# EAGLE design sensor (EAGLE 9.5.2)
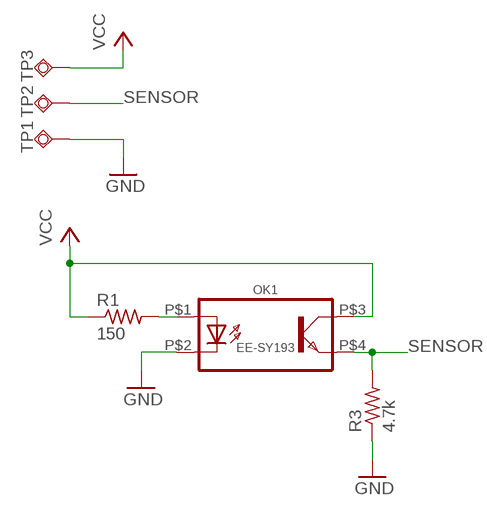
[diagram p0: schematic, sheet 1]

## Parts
OK1  EE-SY193  [EE-SY193]
R1  150  R1206FAB  [R1206FAB]
R3  4.7k  R1206FAB  [R1206FAB]
TP1  TPSQTP14SQ  [TP14SQ]
TP2  TPSQTP14SQ  [TP14SQ]
TP3  TPSQTP14SQ  [TP14SQ]

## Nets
GND: OK1.P$2(C) R3.1 TP1.TP
N$1: OK1.P$1(A) R1.2
SENSOR: OK1.P$4(EMIT) R3.2 TP2.TP
VCC: OK1.P$3(COL) R1.1 TP3.TP

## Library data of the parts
OK1 = EE-SY193:EE-SY193: Photomicrosensor (Reflective); AVAILABILITY: Unavailable; DESCRIPTION: Reflective Optical Sensor 0.039 _1mm_ 4-SMD, No Lead; MF: Omron Electronics; MP: EE-SY193; PACKAGE: SMD-4 Omron; PRICE: None
R1 R3 = eagle_fab:R: Resistor (US Symbol)
TP1-TP3 = testpad:TPSQ: Test pad

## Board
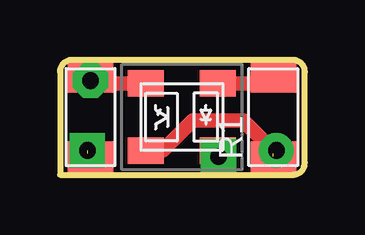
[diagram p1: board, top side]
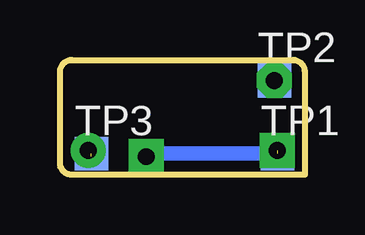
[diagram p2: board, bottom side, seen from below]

Size 10.2 x 4.8 mm. Coordinates in mm from the lower left corner, seen from the top.
Outline: 0,0 9.7,0 arc90 10.2,0.5 10.2,4.3 arc90 9.7,4.8 0.5,4.8 arc90 0,4.3 0,0
Copper layers (1*16): Top 0.035mm / dielectric 1.5mm / Bottom 0.035mm
Design rules "OthermillDRC_1_64_v2": minimum track width 16mil, minimum drill 31mil, track to track 0.39878125mm, track to pad 0.39878125mm, pad to pad 0.39878125mm, via to via 0.39878125mm, smd to smd 0mil, copper to edge 0mil, drill to drill 1mil, minimum pad ring 0mil, minimum via ring 15mil, stop-mask expansion 1mil, vias tented up to drill 30mil, thermal gap 10mil

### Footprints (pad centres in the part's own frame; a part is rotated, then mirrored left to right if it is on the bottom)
EE-SY193 = smd 1.5 x 1.1: P$1 1.5,1.4; P$2 1.5,-1.4; P$3 -1.5,-1.4; P$4 -1.5,1.4
R1206FAB = smd 1.27 x 1.905: 1 -1.651,0; 2 1.651,0
TP14SQ = smd 1.4 x 1.4: TP 0,0

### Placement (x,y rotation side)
OK1  5.08,2.41 0 top
R1  8.89,2.41 90 top
R3  1.27,2.41 90 top
TP1  1.14,0.89 0 bottom
TP2  1.27,3.94 0 bottom
TP3  8.89,0.89 0 bottom

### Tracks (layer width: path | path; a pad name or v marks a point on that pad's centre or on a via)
GND  (via drill 0.7)  (1 unrouted)
  Top 0.61: v1.14,1.02 TP1.TP R3.1 | OK1.P$2 6.6,0.99 v6.6,0.76
  Bottom 0.61: TP1.TP 6.48,0.89 v6.6,0.76
N$1
  Top 0.61: OK1.P$1 8.64,3.81 R1.2
SENSOR  (via drill 0.7)
  Top 0.61: OK1.P$4 1.52,3.81 R3.2 TP2.TP
  other vias: 1.27,3.94
VCC  (via drill 0.7)  (1 unrouted)
  Top 0.61: 8.03,1.85 7.62,2.27 | 7.62,2.27 5.54,2.27 4.29,1.01 OK1.P$3 | v9.02,1.02 TP3.TP R1.1 8.89,1.02 7.64,2.27 7.62,2.27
